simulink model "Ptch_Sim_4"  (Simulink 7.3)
settings: Solver=ode45  StartTime=0.0  StopTime=250  RelTol=1e-3
InitFcn:
  | d2r= pi/180; r2d=1/d2r;
  | [Acl, Bcl, Ccl, Dcl]= closed_loop;    % Load Closed Loop Pitch System
StopFcn:
  | Pl
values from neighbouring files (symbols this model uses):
  Acl = [    [closed_loop.m]
  Bcl = [    [closed_loop.m]
  Ccl = [    [closed_loop.m]
  Dcl = [    [closed_loop.m]

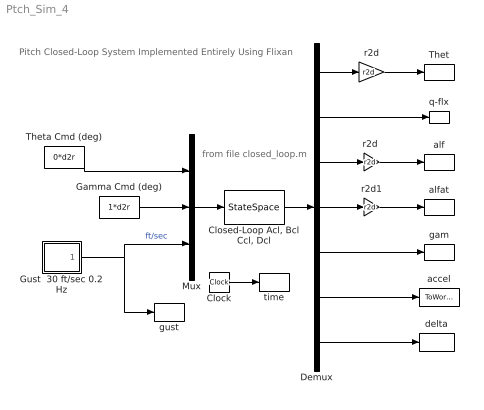
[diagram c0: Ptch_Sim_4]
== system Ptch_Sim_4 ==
  note: Pitch Closed-Loop System Implemented Entirely Using Flixan
  note: from file closed_loop.m
  Clock : Clock
  "Closed-Loop Acl, Bcl Ccl, Dcl" : StateSpace  A=Acl  B=Bcl  C=Ccl  D=Dcl
  Demux : Demux  Outputs=7
  Gamma Cmd (deg) : Constant  Value=1*d2r  OutDataType=sfix(16)  OutScaling=2^0
  Gust  30 ft/sec 0.2 Hz : Subsystem
  Mux : Mux  Inputs=3
  Thet : ToWorkspace  VariableName=theta  SampleTime=-1  SaveFormat=Array
  Theta Cmd (deg) : Constant  Value=0*d2r  OutDataType=sfix(16)  OutScaling=2^0
  accel : ToWorkspace  VariableName=accel  SampleTime=-1  SaveFormat=Array
  alf : ToWorkspace  VariableName=alpha  SampleTime=-1  SaveFormat=Array
  alfat : ToWorkspace  VariableName=alphat  SampleTime=-1  SaveFormat=Array
  delta : ToWorkspace  VariableName=delta  SampleTime=-1  SaveFormat=Array
  gam : ToWorkspace  VariableName=gama  SampleTime=-1  SaveFormat=Array
  gust : ToWorkspace  VariableName=Gust  SampleTime=-1  SaveFormat=Array
  q-flx : ToWorkspace  VariableName=q  SampleTime=-1  SaveFormat=Array
  r2d : Gain  Gain=r2d  ParameterDataType=sfix(16)  ParameterScaling=2^0  OutDataType=sfix(16)  OutScaling=2^0
  "r2d " : Gain  Gain=r2d  ParameterDataType=sfix(16)  ParameterScaling=2^0  OutDataType=sfix(16)  OutScaling=2^0
  r2d1 : Gain  Gain=r2d  ParameterDataType=sfix(16)  ParameterScaling=2^0  OutDataType=sfix(16)  OutScaling=2^0
  time : ToWorkspace  VariableName=time  SampleTime=-1  SaveFormat=Array
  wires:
  Mux/1 -> "Closed-Loop Acl, Bcl Ccl, Dcl"/1
  Demux/6 -> accel/1
  Demux/5 -> gam/1
  Clock/1 -> time/1
  r2d/1 -> Thet/1
  "r2d "/1 -> alf/1
  Theta Cmd (deg)/1 -> Mux/1
  Gust  30 ft/sec 0.2 Hz/1(Vgust) -> Mux/3, gust/1  "ft/sec"
  Gamma Cmd (deg)/1 -> Mux/2
  "Closed-Loop Acl, Bcl Ccl, Dcl"/1 -> Demux/1
  Demux/1 -> r2d/1
  Demux/2 -> q-flx/1
  Demux/3 -> "r2d "/1
  Demux/4 -> r2d1/1
  r2d1/1 -> alfat/1
  Demux/7 -> delta/1

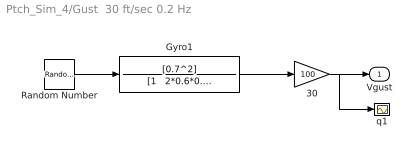
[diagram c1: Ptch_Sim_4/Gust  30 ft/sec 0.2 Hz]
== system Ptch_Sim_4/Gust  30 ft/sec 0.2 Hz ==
  30 : Gain  Gain=100  ParameterDataType=sfix(16)  ParameterScaling=2^0  OutDataType=sfix(16)  OutScaling=2^0
  Gyro1 : TransferFcn  Numerator=[0.7^2]  Denominator="[1   2*0.6*0.7   0.7^2]"
  Random Number : RandomNumber  Seed=-2  SampleTime=0
  q1 : Scope
  Vgust : Outport  OutDataType=sfix(16)  OutScaling=2^0
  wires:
  30/1 -> q1/1, Vgust/1
  Gyro1/1 -> 30/1
  Random Number/1 -> Gyro1/1
